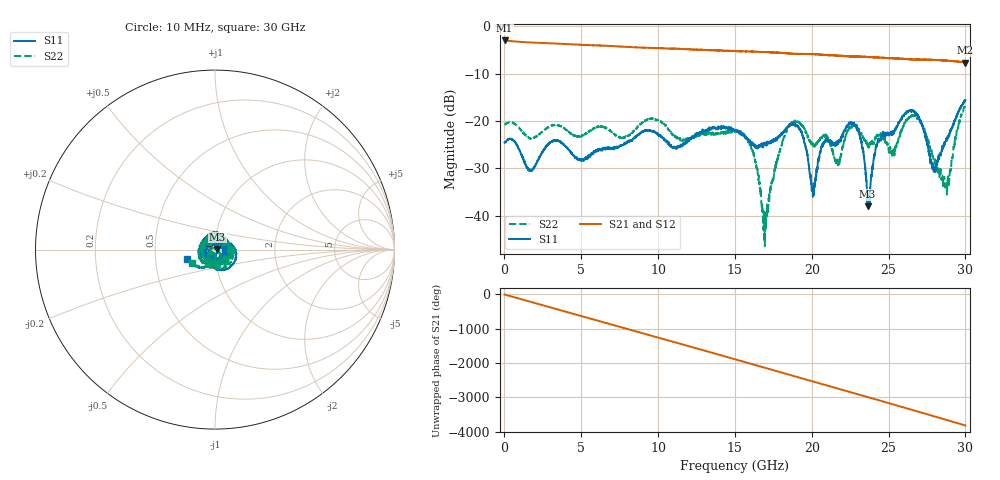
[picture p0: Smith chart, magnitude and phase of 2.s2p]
#  HZ  S  DB  R  50.00
! Rohde & Schwarz Vector Network Analyzer
! Rohde-Schwarz,ZNB40-4Port,1311601084101679,3.45
! Created: UTC 10/20/2022, 5:23:28 PM
! freq[Hz]  db:S11  ang:S11  db:S31  ang:S31  db:S13  ang:S13  db:S33  ang:S33
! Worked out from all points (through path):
!   3000 points, 10 MHz to 30 GHz, reference 50 ohm
!   highest |S21| = -2.98 dB at 10 MHz (marker M1); lowest = -7.7 dB at 30 GHz (marker M2)
!   group delay of S21, straight-line fit = 353 ps
!   lowest |S11| = -38.0 dB at 23.63 GHz (marker M3), VSWR 1.03, Z = 51.2 + j0.377 ohm
!   |S11| at or under -10 dB: start of sweep to end of sweep
!   |S22| runs from -46.4 to -16.5 dB; largest |S21 - S12| = 0.0084
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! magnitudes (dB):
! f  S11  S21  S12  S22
! 10 MHz  -24.5  -3.0  -3.0  -20.8
! 1.68 GHz  -30.5  -3.4  -3.4  -23.7
! 3.28 GHz  -24.1  -3.6  -3.6  -20.8
! 5.01 GHz  -28.2  -3.9  -3.9  -23.1
! 10.01 GHz  -22.9  -4.6  -4.6  -19.8
! 15.01 GHz  -21.9  -5.2  -5.2  -22.3
! 16.13 GHz  -24.8  -5.4  -5.3  -26.1
! 16.93 GHz  -24.8  -5.4  -5.5  -43.0
! 18.55 GHz  -21.1  -5.7  -5.7  -21.0
! 19.34 GHz  -22.6  -5.8  -5.8  -20.8
! 20.01 GHz  -34.0  -5.9  -5.9  -24.5
! 20.77 GHz  -24.8  -6.0  -6.0  -23.2
! 21.7 GHz  -24.6  -6.2  -6.1  -29.1
! 22.6 GHz  -20.3  -6.3  -6.4  -21.4
! 23.22 GHz  -24.3  -6.4  -6.4  -22.5
! 23.63 GHz  -38.0  -6.5  -6.4  -25.3
! 24.29 GHz  -24.4  -6.6  -6.5  -23.0
! 25.01 GHz  -23.0  -6.7  -6.7  -26.2
! 26.79 GHz  -18.4  -7.0  -7.0  -19.1
! 27.96 GHz  -30.5  -7.1  -7.0  -29.0
! 28.79 GHz  -24.2  -7.2  -7.2  -34.0
! 30 GHz  -15.7  -7.7  -7.6  -16.5
